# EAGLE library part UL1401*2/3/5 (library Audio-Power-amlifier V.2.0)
Polish CEMI UL1401,UL1402,UL1403,UL1405
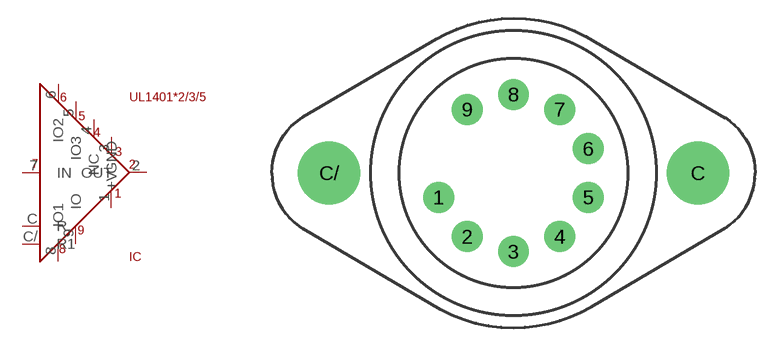
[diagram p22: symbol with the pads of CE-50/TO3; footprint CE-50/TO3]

Designator prefix IC

## UL14012/3/5  [CE-50/TO3]
1  GND  pwr
2  OUT  out
3  +V  pwr
4  NC
5  IO3
6  IO2
7  IN  in
8  IO1
9  IO
C  R  pwr
C/  R1  pwr

## Footprint CE-50/TO3 (pad centres in mm)
TO-3 National Semiconductor K08A
drill 1 pad 2.54: 1 -6.134,-1.993; 2 -3.791,-5.218; 3 0,-6.45; 4 3.791,-5.218; 5 6.134,-1.993; 6 6.134,1.993; 7 3.791,5.218; 8 0,6.45; 9 -3.791,5.218
drill 4.115: C 15.113,0; C/ -15.113,0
